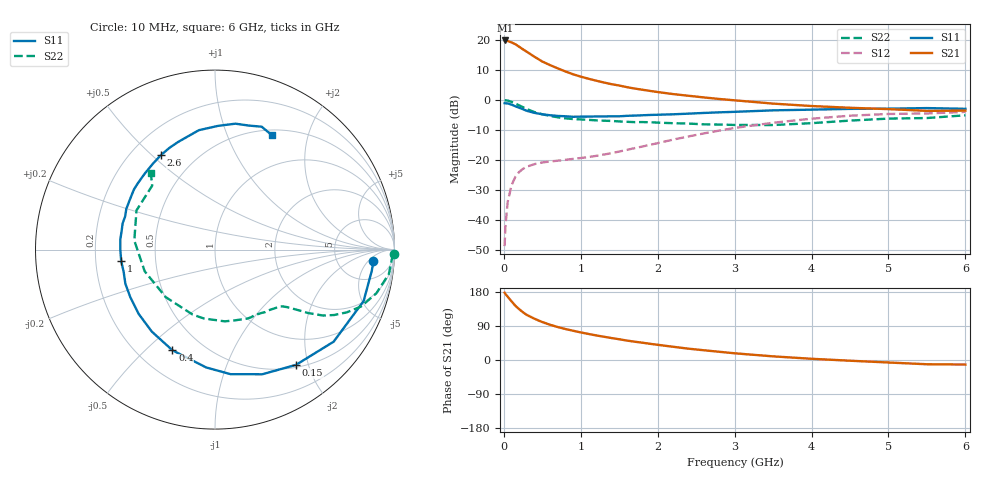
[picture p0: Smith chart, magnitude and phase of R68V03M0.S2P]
! SIEMENS Small Signal Semiconductors
! BFR193
! Si NPN RF Bipolar Junction Transistor in SOT23
! VCE = 8 V  IC = 3 mA
! Common Emitter S-Parameters:  May  1996
# GHz  S  MA  R  50
!  f  S11  S21  S12  S22
! GHz  MAG  ANG  MAG  ANG  MAG  ANG  MAG  ANG
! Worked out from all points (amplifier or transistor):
!   36 points, 10 MHz to 6 GHz, reference 50 ohm
!   highest |S21| = 19.9 dB at 20 MHz (marker M1)
!   |S21| within 3 dB of that: start of sweep to 250.7 MHz
!   unconditionally stable (mu >= 1): 1.067 GHz to 2.032 GHz
!   at 250 MHz: K = 0.30, MSG = 20.0 dB, |S12| = -23.0 dB
!   at 1.4 GHz: K = 1.08, MAG = 9.8 dB, |S12| = -17.8 dB
!   at 6 GHz: K = 0.98, MSG = 0.2 dB, |S12| = -4.0 dB
!   S11 on the Smith chart (normalised r, x): 10 MHz: 12, -7; 150 MHz: 0.54, -1.80; 400 MHz: 0.34, -0.61; 1 GHz: 0.31, -0.05; 2.6 GHz: 0.32, +0.54; 6 GHz: 0.56, +1.46
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0.01  0.8853 -4.1  9.747 177.6  0.0036 86.2  0.9949 -1.5
0.02  0.8814 -7.8  9.895 174.5  0.0075 85.9  0.9864 -3.2
0.05  0.8762 -19.1  9.698 167.0  0.0197 79.0  0.9782 -8.0
0.1  0.8368 -37.8  9.172 154.9  0.0376 70.0  0.9318 -15.1
0.15  0.7849 -54.9  8.558 143.0  0.0521 62.3  0.8734 -21.3
0.2  0.7429 -69.2  7.751 134.0  0.0628 56.2  0.8128 -25.5
0.25  0.6998 -82.8  7.014 125.7  0.0709 51.2  0.7567 -28.8
0.3  0.6584 -94.3  6.387 118.8  0.077 47.7  0.7051 -31.4
0.4  0.6091 -112.9  5.265 108.7  0.0848 43.0  0.6268 -34.3
0.5  0.5768 -127.6  4.395 100.1  0.0903 40.7  0.5768 -35.9
0.6  0.5561 -139.9  3.835 93.1  0.0938 39.9  0.5419 -37.3
0.7  0.5415 -150.5  3.386 87.0  0.0966 40.7  0.5138 -38.6
0.8  0.5343 -159.2  3.003 81.8  0.1 41.7  0.4937 -39.9
1  0.5264 -173.3  2.46 72.8  0.1072 45.1  0.4735 -42.8
1.1  0.5277 179.9  2.265 68.8  0.1114 47.4  0.4651 -44.9
1.6  0.5437 155.3  1.639 51.3  0.1466 57.3  0.4322 -56.2
2.2  0.5766 132.8  1.256 34.9  0.2177 60.9  0.4092 -74.6
2.6  0.6074 119.5  1.104 25.7  0.2765 58.5  0.392 -90.3
3.5  0.6714 97.7  0.87 9.6  0.4166 45.4  0.3814 -136.0
4.5  0.7107 80.8  0.741 -1.9  0.5462 26.6  0.4524 173.6
5.5  0.7325 69.2  0.658 -11.2  0.5958 7.9  0.4994 134.5
6  0.7124 63.7  0.665 -12.0  0.6327 2.7  0.5551 130.1
